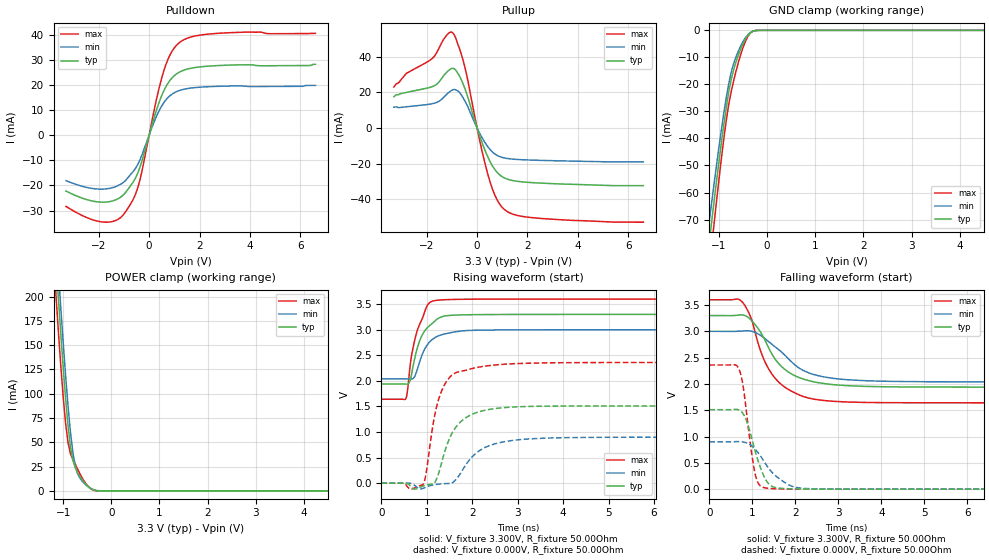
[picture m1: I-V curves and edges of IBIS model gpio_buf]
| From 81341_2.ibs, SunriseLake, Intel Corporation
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[Model]   gpio_buf
Model_type   I/O
Vinl = 1.155V
Vinh = 1.650V
Vmeas = 1V
Vref = 0.000V
Cref = 10.000pF
Rref = 100.000Ohm
|   typ   min   max
C_comp   5.000pF   4.750pF   5.250pF
[Voltage Range]   3.300V   3.000V   3.600V
[Temperature Range]   60.0   110.0   -5.0
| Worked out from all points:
|   slope of the pulldown table from 0 to 0.495 V, typ, clamps not added: 31.4 ohm
|   slope of the pullup table from 0 to 0.495 V, typ, clamps not added: 27.1 ohm
|   GND clamp passes 1 mA (typ) near -0.35 V on its own axis
|   POWER clamp passes 1 mA (typ) near -0.36 V on its own axis
|   falling waveform, V_fixture 3.300V, R_fixture 50.00Ohm: 20-80 % time 711ps typ, 878ps min, 628ps max; typ from 3.3 V to 1.94 V
|   rising waveform, V_fixture 3.300V, R_fixture 50.00Ohm: 20-80 % time 317ps typ, 325ps min, 293ps max; typ from 1.94 V to 3.3 V
|   rising waveform, V_fixture 0.000V, R_fixture 50.00Ohm: 20-80 % time 460ps typ, 603ps min, 339ps max; typ from 0 V to 1.51 V
|   falling waveform, V_fixture 0.000V, R_fixture 50.00Ohm: 20-80 % time 338ps typ, 554ps min, 225ps max; typ from 1.51 V to 0 V
[Pulldown]
|   Voltage   I(typ)   I(min)   I(max)
-3.3V     -22.26mA   -18.1mA    -28.36mA
-1.85V    -26.68mA   -21.46mA   -34.58mA
-1.35V    -25.84mA   -20.55mA   -34.06mA
-950mV    -22.96mA   -18.12mA   -30.7mA
-600mV    -18.08mA   -14mA      -24.85mA
-400mV    -13.72mA   -10.54mA   -19.12mA
300mV     10.36mA    7.775mA    14.76mA
600mV     18.11mA    13.26mA    26.28mA
900mV     22.81mA    16.36mA    33.4mA
1.25V     25.45mA    18.04mA    37.35mA
2.7V      27.81mA    19.53mA    40.66mA
6.6V      28.32mA    19.91mA    40.67mA
[GND Clamp]
|   Voltage   I(typ)   I(min)   I(max)
-3.3V     -392.6mA   -362.9mA   -431.7mA
-1.25V    -85.75mA   -77.5mA    -96.38mA
-1.2V     -78.06mA   -70.39mA   -87.87mA
-1.15V    -70.46mA   -63.37mA   -79.46mA
-1.1V     -62.97mA   -56.47mA   -71.17mA
-900mV    -34.89mA   -30.68mA   -40.16mA
-750mV    -18.5mA    -15.77mA   -23mA
-650mV    -11.89mA   -9.961mA   -15.39mA
-500mV    -4.899mA   -4.134mA   -6.303mA
-400mV    -1.867mA   -1.637mA   -2.26mA
-300mV    -357.3uA   -362.2uA   -330uA
6.6V      0A         0A         0A
[Pullup]
|   Voltage   I(typ)   I(min)   I(max)
-3.3V     17.54mA    11.64mA    22.96mA
-1.7V     23.63mA    13.85mA    40.08mA
-1.3V     29.73mA    17.56mA    50.22mA
-1V       33.32mA    21.11mA    53.64mA
-850mV    32.44mA    21.41mA    50.53mA
-500mV    22.7mA     15.56mA    34.96mA
100mV     -4.257mA   -2.852mA   -6.724mA
450mV     -16.93mA   -10.96mA   -27.09mA
750mV     -24.13mA   -15.01mA   -39mA
1.05V     -27.75mA   -16.72mA   -45.25mA
2.1V      -30.57mA   -17.98mA   -50.15mA
6.6V      -32.35mA   -19.06mA   -52.81mA
[POWER Clamp]
|   Voltage   I(typ)   I(min)   I(max)
-3.3V     1.906A     1.939A     1.845A
-1.15V    237.5mA    264.5mA    202.2mA
-1.1V     199.5mA    226.3mA    164.9mA
-1.05V    162.8mA    189.2mA    129.5mA
-950mV    95.69mA    119.4mA    69.99mA
-900mV    67.74mA    88.25mA    50.02mA
-850mV    45.99mA    61.3mA     38.57mA
-800mV    32.08mA    40.38mA    32.57mA
-750mV    24.08mA    25.9mA     27.87mA
-700mV    18.75mA    17.74mA    22.46mA
-400mV    1.715mA    1.884mA    1.374mA
6.6V      0A         0A         0A
[Ramp]
R_load = 50.00Ohm
|   typ   min   max
dV/dt_r   906.362mV/458.345ps 539.525mV/602.578ps   1.416V/338.643ps
dV/dt_f   816.291mV/710.575ps 576.548mV/875.957ps   1.175V/627.483ps
[Falling Waveform]
V_fixture = 3.300V
V_fixture_min = 3.000V
V_fixture_max = 3.600V
R_fixture = 50.00Ohm
|   Time   V(typ)   V(min)   V(max)
0s        3.3V       3V         3.6V
760ps     3.313V     3.005V     3.562V
950ps     3.232V     3.007V     3.293V
1.09ns    3.101V     2.97V      2.902V
1.25ns    2.901V     2.888V     2.501V
1.45ns    2.575V     2.757V     2.194V
1.79ns    2.254V     2.519V     1.92V
2.31ns    2.063V     2.211V     1.732V
4.01ns    1.947V     2.052V     1.645V
10.3ns    1.94V      2.039V     1.641V
[Rising Waveform]
V_fixture = 3.300V
V_fixture_min = 3.000V
V_fixture_max = 3.600V
R_fixture = 50.00Ohm
|   Time   V(typ)   V(min)   V(max)
0s        1.94V      2.039V     1.641V
540ps     1.938V     2.039V     1.658V
570ps     1.936V     2.039V     1.785V
630ps     2.006V     2.037V     2.286V
770ps     2.579V     2.171V     2.929V
1ns       3.03V      2.693V     3.458V
1.16ns    3.158V     2.836V     3.568V
1.42ns    3.273V     2.924V     3.588V
2.12ns    3.296V     2.992V     3.598V
10.3ns    3.3V       3V         3.6V
[Rising Waveform]
V_fixture = 0.000V
V_fixture_min = 0.000V
V_fixture_max = 0.000V
R_fixture = 50.00Ohm
|   Time   V(typ)   V(min)   V(max)
0s        450.3nV    3.1uV      28.16nV
920ps     -54.25mV   -99.64mV   -19.8mV
980ps     -38.39mV   -77.42mV   178.1mV
1.15ns    -9.942mV   -31.6mV    1.222V
1.27ns    225.5mV    -16.86mV   1.671V
1.47ns    814.6mV    -5.55mV    2.037V
1.7ns     1.162V     139.8mV    2.179V
2.17ns    1.402V     643.6mV    2.274V
3.02ns    1.495V     849.6mV    2.34V
10.3ns    1.511V     899.2mV    2.36V
[Falling Waveform]
V_fixture = 0.000V
V_fixture_min = 0.000V
V_fixture_max = 0.000V
R_fixture = 50.00Ohm
|   Time   V(typ)   V(min)   V(max)
0s        1.511V     899.2mV    2.36V
690ps     1.505V     903.2mV    2.28V
790ps     1.427V     895.1mV    1.93V
970ps     1.013V     832.3mV    761mV
1.06ns    738.7mV    764.8mV    306.7mV
1.14ns    522.3mV    685.4mV    108.6mV
1.27ns    244.3mV    529.6mV    29.58mV
1.5ns     38.82mV    283.9mV    8.994mV
2.19ns    3.096mV    14.77mV    857.7uV
10.3ns    450.3nV    3.1uV      28.16nV
